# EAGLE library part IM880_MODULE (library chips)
Lora Radio module by IMST
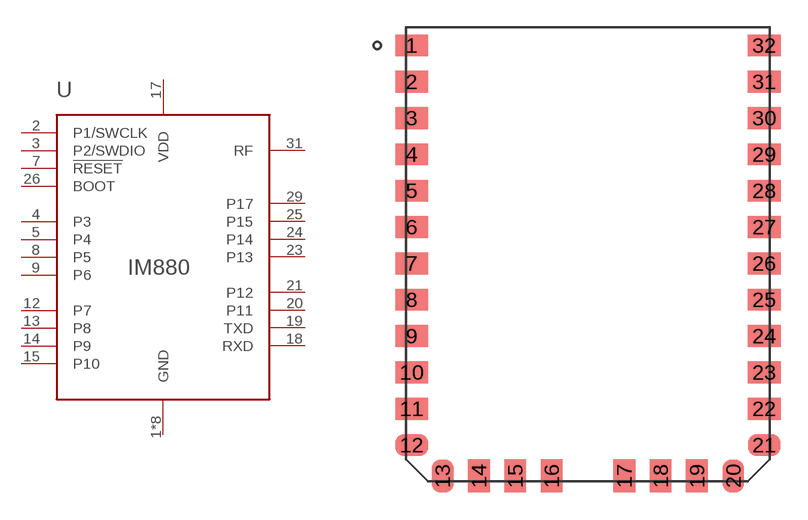
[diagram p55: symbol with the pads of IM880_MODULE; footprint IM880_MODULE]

Designator prefix U

## IM880_MODULE  [IM880_MODULE]
1  GND
2  P1/SWCLK
3  P2/SWDIO
4  P3
5  P4
6  GND
7  !RESET
8  P5
9  P6
11  GND
12  P7
13  P8
14  P9
15  P10
16  GND
17  VDD
18  RXD
19  TXD
20  P11
21  P12
22  GND
23  P13
24  P14
25  P15
26  BOOT
27  GND
29  P17
30  GND
31  RF
32  GND

## Footprint IM880_MODULE (pad centres in mm)
smd 1.8 x 1.2: 1 -9.7,11; 2 -9.7,9; 3 -9.7,7; 4 -9.7,5; 5 -9.7,3; 6 -9.7,1; 7 -9.7,-1; 8 -9.7,-3; 9 -9.7,-5; 10 -9.7,-7; 11 -9.7,-9; 12 -9.7,-11; 21 9.7,-11; 22 9.7,-9; 23 9.7,-7; 24 9.7,-5; 25 9.7,-3; 26 9.7,-1; 27 9.7,1; 28 9.7,3; 29 9.7,5; 30 9.7,7; 31 9.7,9; 32 9.7,11
smd 1.2 x 1.8: 13 -8,-12.7; 14 -6,-12.7; 15 -4,-12.7; 16 -2,-12.7; 17 2,-12.7; 18 4,-12.7; 19 6,-12.7; 20 8,-12.7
